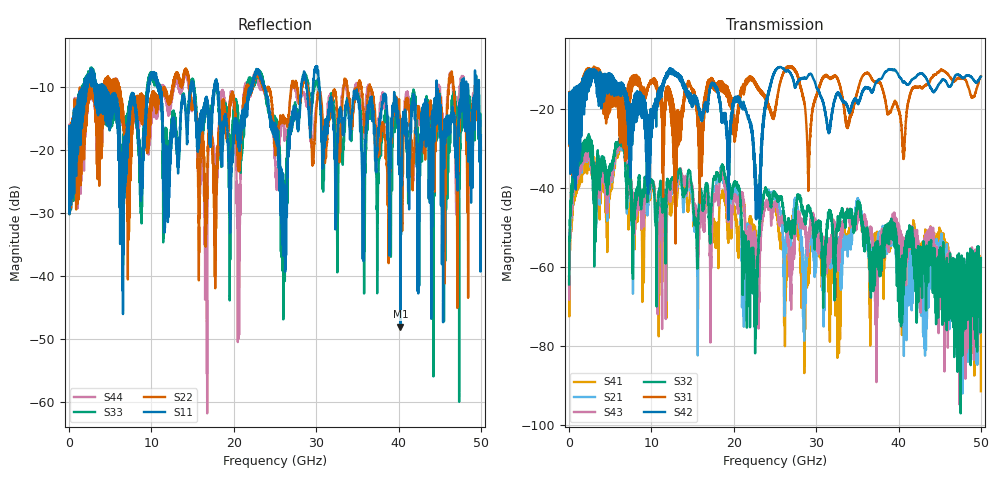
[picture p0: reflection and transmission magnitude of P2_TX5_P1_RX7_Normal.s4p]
!Keysight Technologies,N5225B,MY57041031,A.13.20.10
!Date: Friday, May 31, 2019 11:25:14
!Correction: S11(Full 4 Port(1,2,3,4))
!S12(Full 4 Port(1,2,3,4))
!S13(Full 4 Port(1,2,3,4))
!S14(Full 4 Port(1,2,3,4))
!S21(Full 4 Port(1,2,3,4))
!S22(Full 4 Port(1,2,3,4))
!S23(Full 4 Port(1,2,3,4))
!S24(Full 4 Port(1,2,3,4))
!S31(Full 4 Port(1,2,3,4))
!S32(Full 4 Port(1,2,3,4))
!S33(Full 4 Port(1,2,3,4))
!S34(Full 4 Port(1,2,3,4))
!S41(Full 4 Port(1,2,3,4))
!S42(Full 4 Port(1,2,3,4))
!S43(Full 4 Port(1,2,3,4))
!S44(Full 4 Port(1,2,3,4))
!S4P File: Measurements: <S11,S12,S13,S14>,
!<S21,S22,S23,S24>,
!<S31,S32,S33,S34>,
!<S41,S42,S43,S44>:
# Hz S  dB  R 50.0
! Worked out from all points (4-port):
!   5000 points, 10 MHz to 50 GHz, reference 50 ohm
!   strongest paths, dB at 10 MHz, 12.51 GHz, 25.01 GHz, 37.51 GHz, 50 GHz:
!     S42: -19.6, -9.9, -10.6, -12.7, -11.8
!     S31: -19.4, -17.8, -20.9, -13.2, -11.8
!     S32: -64.3, -37.3, -41.6, -53.9, -57.7
!     S43: -62.3, -39.3, -44.0, -57.5, -66.3
!     S21: -62.2, -40.2, -43.0, -52.0, -74.8
!     S41: -62.3, -44.1, -45.0, -55.4, -91.3
!   lowest |S11| = -48.0 dB at 40.22 GHz (marker M1), VSWR 1.01, Z = 49.6 + j0.144 ohm
!   |S11| at or under -10 dB: 4.421 GHz to 9.567 GHz (5.146 GHz wide, 73.6 % of centre); 23.74 GHz to 28.17 GHz (4.438 GHz wide, 17.1 % of centre); 30.39 GHz to 44.6 GHz (14.21 GHz wide, 37.9 % of centre)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
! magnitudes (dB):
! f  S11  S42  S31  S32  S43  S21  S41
! 10 MHz  -18.9  -19.6  -19.4  -64.3  -62.3  -62.2  -62.3
! 6.36 GHz  -24.3  -15.7  -16.3  -29.3  -29.5  -30.3  -30.5
! 16.61 GHz  -13.9  -19.1  -16.0  -39.0  -42.2  -39.5  -42.4
! 22.93 GHz  -7.1  -39.6  -14.9  -59.0  -64.5  -56.1  -58.3
! 25.32 GHz  -19.1  -9.6  -16.7  -42.7  -45.9  -43.5  -47.7
! 40.22 GHz  -48.0  -12.1  -22.0  -62.0  -51.9  -57.7  -61.1
! 50 GHz  -20.4  -11.8  -11.8  -57.7  -66.3  -74.8  -91.3
